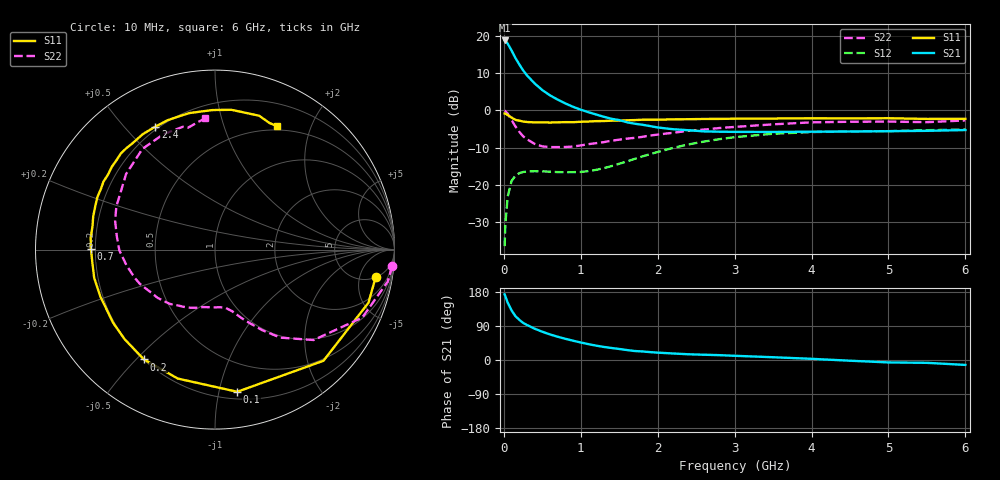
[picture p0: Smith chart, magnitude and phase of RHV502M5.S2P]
! SIEMENS Small Signal Semiconductors
! BFR106
! Si NPN RF Bipolar Junction Transistor in SOT23
! VCE = 0.5 V  IC = 2.5 mA
! Common Emitter S-Parameters:  August  1996
# GHz  S  MA  R  50
!  f  S11  S21  S12  S22
! GHz  MAG  ANG  MAG  ANG  MAG  ANG  MAG  ANG
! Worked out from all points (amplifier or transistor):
!   36 points, 10 MHz to 6 GHz, reference 50 ohm
!   highest |S21| = 18.8 dB at 10 MHz (marker M1)
!   |S21| within 3 dB of that: start of sweep to 108.1 MHz
!   unconditionally stable (mu >= 1): 691.2 MHz to end of sweep
!   at 250 MHz: K = 0.39, MSG = 13.6 dB, |S12| = -16.5 dB
!   at 1.4 GHz: K = 1.34, MAG = 2.8 dB, |S12| = -14.9 dB
!   at 6 GHz: K = 1.03, MAG = -1.1 dB, |S12| = -5.1 dB
!   S11 on the Smith chart (normalised r, x): 10 MHz: 5, -9; 100 MHz: 0.26, -1.14; 200 MHz: 0.20, -0.53; 700 MHz: 0.18, +0.00; 2.4 GHz: 0.19, +0.61; 6 GHz: 0.46, +1.53
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0.01  0.9082 -9.7  8.668 173.3  0.0151 85.5  0.991 -5.4
0.02  0.9048 -19.1  8.573 168.2  0.0299 80.5  0.9787 -10.5
0.05  0.8654 -45.7  7.853 151.3  0.0696 64.4  0.9037 -24.8
0.1  0.8018 -81.1  6.371 131.0  0.1126 47.3  0.7456 -42.5
0.15  0.7478 -106.1  5.055 115.9  0.1334 36.0  0.611 -53.4
0.2  0.7287 -122.9  4.154 106.2  0.1438 29.5  0.5181 -59.8
0.25  0.709 -135.3  3.448 98.1  0.1491 24.8  0.4501 -65.0
0.3  0.699 -144.3  2.955 92.4  0.1515 22.3  0.4113 -68.6
0.4  0.6903 -157.7  2.3 82.7  0.153 19.0  0.3553 -74.6
0.5  0.6913 -166.9  1.871 74.6  0.1521 17.9  0.3294 -79.8
0.6  0.6872 -174.5  1.592 67.5  0.1507 18.1  0.3222 -84.9
0.7  0.6915 179.5  1.394 61.4  0.1487 19.3  0.3221 -90.8
0.9  0.6947 169.3  1.117 50.9  0.1484 24.5  0.3272 -101.9
1.1  0.7093 160.2  0.945 41.8  0.1534 31.6  0.3523 -113.2
1.6  0.7369 141.3  0.693 26.3  0.207 45.1  0.418 -140.1
2.2  0.7587 121.9  0.559 17.2  0.314 43.9  0.501 -170.0
2.4  0.7615 115.9  0.542 15.1  0.3496 40.9  0.5329 -179.5
3.5  0.7777 90.9  0.514 7.3  0.4856 20.4  0.65 139.7
4.5  0.7809 77.2  0.521 -1.9  0.5215 4.3  0.7038 114.3
5  0.7853 71.7  0.526 -6.4  0.527 -1.7  0.7075 104.7
5.5  0.7681 66.8  0.532 -7.5  0.5421 -4.6  0.6956 102.5
6  0.7695 63.1  0.545 -13.0  0.5555 -11.1  0.7337 94.4
